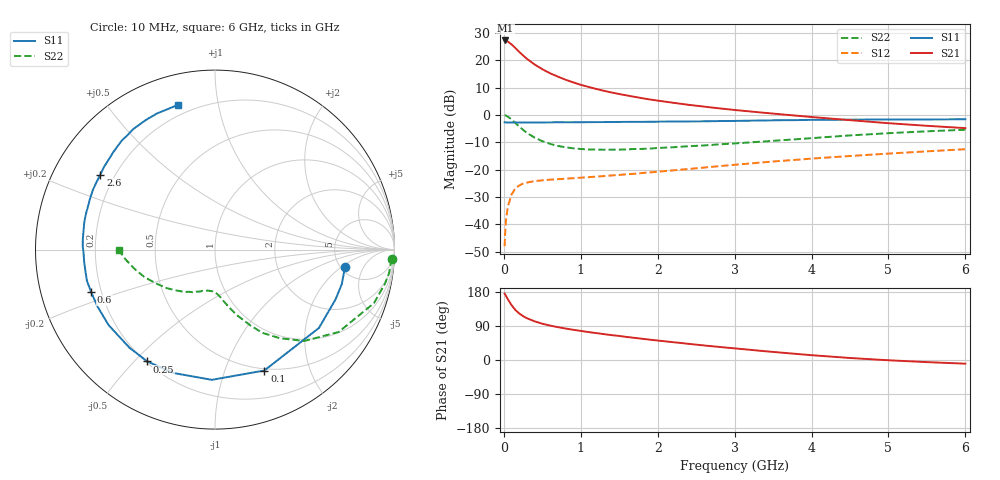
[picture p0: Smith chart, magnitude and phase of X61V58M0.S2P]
! SIEMENS Small Signal Semiconductors
! BFP193W
! Si NPN RF Bipolar Junction Transistor in SOT343
! VCE = 1.5 V  IC = 8 mA
! Common Emitter S-Parameters:  April 1994
# GHz  S  MA  R  50
!  f  S11  S21  S12  S22
! GHz  MAG  ANG  MAG  ANG  MAG  ANG  MAG  ANG
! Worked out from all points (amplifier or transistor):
!   40 points, 10 MHz to 6 GHz, reference 50 ohm
!   highest |S21| = 27.2 dB at 20 MHz (marker M1)
!   |S21| within 3 dB of that: start of sweep to 158.3 MHz
!   unconditionally stable (mu >= 1): 1.378 GHz to 4.464 GHz
!   at 200 MHz: K = 0.20, MSG = 24.4 dB, |S12| = -25.8 dB
!   at 1.5 GHz: K = 1.04, MAG = 13.5 dB, |S12| = -21.9 dB
!   at 6 GHz: K = 0.94, MSG = 3.8 dB, |S12| = -12.5 dB
!   S11 on the Smith chart (normalised r, x): 10 MHz: 5.48, -2.24; 100 MHz: 0.48, -1.38; 250 MHz: 0.21, -0.55; 600 MHz: 0.16, -0.16; 2.6 GHz: 0.15, +0.29; 6 GHz: 0.15, +0.77
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0.01  0.7307 -7.5  22.87 175.3  0.004 86.7  0.9855 -3.0
0.02  0.7323 -15.2  22.89 172.2  0.0085 83.2  0.9785 -7.8
0.03  0.7267 -22.4  22.66 168.4  0.0125 79.0  0.9654 -11.4
0.05  0.7252 -37.0  21.97 160.9  0.0205 72.7  0.9347 -18.6
0.1  0.7276 -67.8  19.42 144.8  0.0351 59.0  0.8278 -33.7
0.15  0.7258 -91.4  16.65 132.0  0.0454 48.5  0.7116 -45.7
0.2  0.7256 -108.7  14.15 122.7  0.0514 41.7  0.6107 -53.9
0.25  0.7284 -121.2  12.19 115.8  0.0557 37.0  0.5342 -60.3
0.3  0.7253 -131.1  10.56 110.2  0.0581 33.7  0.4685 -64.8
0.4  0.7269 -144.7  8.329 102.0  0.0618 29.8  0.3844 -71.6
0.5  0.7273 -154.1  6.837 95.7  0.0637 28.1  0.3315 -76.2
0.6  0.7298 -161.1  5.769 90.9  0.0655 27.2  0.2959 -80.0
0.8  0.7317 -171.0  4.402 83.1  0.0682 28.0  0.2564 -85.3
1.1  0.7369 178.7  3.248 73.8  0.0728 30.2  0.2334 -92.1
1.3  0.7391 173.2  2.755 68.3  0.0763 32.3  0.2315 -96.3
1.6  0.7453 166.0  2.264 60.7  0.0824 35.3  0.2344 -101.9
2.2  0.7572 154.0  1.666 47.0  0.097 40.1  0.2564 -113.9
2.6  0.7634 146.8  1.418 38.4  0.109 42.0  0.2765 -121.9
3.2  0.7839 136.6  1.156 26.9  0.1296 43.0  0.3143 -133.6
4.5  0.8186 118.1  0.801 5.3  0.1775 39.7  0.4221 -158.7
5.5  0.8256 108.8  0.632 -5.6  0.2159 35.0  0.5012 -173.7
6  0.8325 104.3  0.573 -9.7  0.2362 32.6  0.5359 -179.7
